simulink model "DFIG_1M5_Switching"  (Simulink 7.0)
settings: Solver=ode45  SolverMode=SingleTasking  StartTime=0  StopTime=Tstop  FixedStep=0,000005  MaxStep=0.001  RelTol=1e-3  AbsTol=1e-6
InitFcn:
  | DFIG_init_sw
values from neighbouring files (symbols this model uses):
  gearbox = 75.7098    [DFIG_init_simp.m]    (also in DFIG_init_sw.m)
  ki_i = 0.003    [DFIG_init_simp.m]    (also in DFIG_init_sw.m)
  kp_i = 0.00003    (= 3e-05)    [DFIG_init_simp.m]    (also in DFIG_init_sw.m)
  L = 0.6e-3    (= 0.0006)    [DFIG_init_simp.m]    (also in DFIG_init_sw.m)
  R = 35    [DFIG_init_simp.m]    (also in DFIG_init_sw.m)
  TSR_opt = 8    [DFIG_init_simp.m]    (also in DFIG_init_sw.m)
  Tswitch = 0.2    [DFIG_init_simp.m]    (also in DFIG_init_sw.m)
  Vw1 = 10.5    [DFIG_init_simp.m]    (also in DFIG_init_sw.m)
  Vw2 = 8    [DFIG_init_simp.m]    (also in DFIG_init_sw.m)
  zp = 2    [DFIG_init_simp.m]    (also in DFIG_init_sw.m)
undefined symbols (not defined in the file or in its folder): carrier, Natural, plecsedit, starts, with
libraries: plecslib x10, plecslib_extras x7, simulink x2

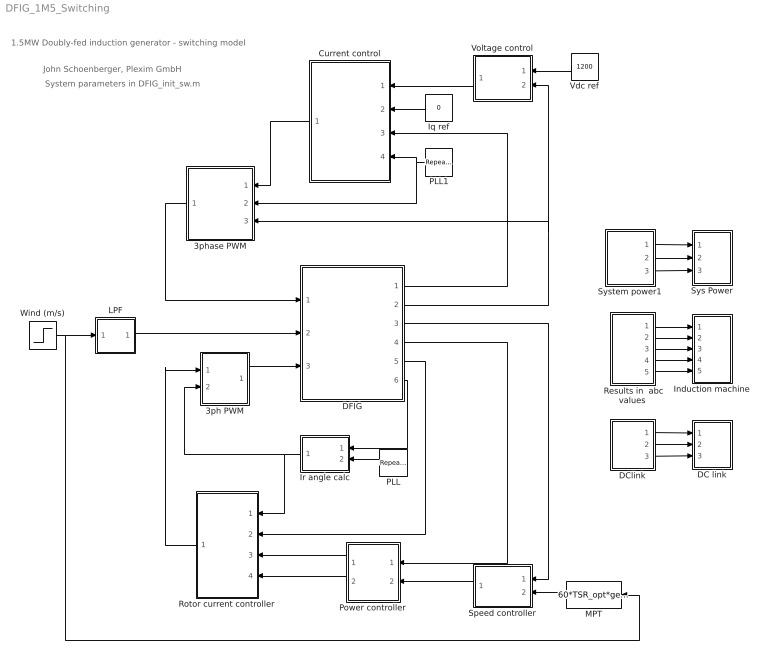
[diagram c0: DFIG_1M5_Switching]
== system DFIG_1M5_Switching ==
  note: John Schoenberger, Plexim GmbH
  note: 1.5MW Doubly-fed induction generator - switching model
  note: System parameters in DFIG_init_sw.m
  " Results in  abc values" : Subsystem
  3ph PWM : Subsystem
  3phase PWM : Subsystem  Orientation=left
  Current control : Subsystem  Orientation=left
  DC link : Subsystem  LoadFcn=plecsedit('sl', 300);  StartFcn=plecsedit('sl', 308);  StopFcn=plecsedit('sl', 309);  mask{Settings=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}
      mask init:
      | plecsedit('sl', 315);
  DClink : Subsystem
  DFIG : Subsystem  LoadFcn=plecsedit('sl', 200);  InitFcn=plecsedit('sl', 214);  StartFcn=plecsedit('sl', 208);  StopFcn=plecsedit('sl', 209);
  Induction machine : Subsystem  LoadFcn=plecsedit('sl', 300);  StartFcn=plecsedit('sl', 308);  StopFcn=plecsedit('sl', 309);  mask{Settings=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}
      mask init:
      | plecsedit('sl', 315);
  Iq ref : Constant  Orientation=left  Value=0  OutDataType=sfix(16)  OutScaling=2^0
  Ir angle calc : Subsystem  Orientation=left
  LPF : Subsystem  mask{tau=0.2, y0=Vw1}
      mask prompts: tau "Time constant"; y0 "Initial output"
  MPT : Fcn  Orientation=left  Expr=60*TSR_opt*gearbox*u(1)/(2*pi*R)
  PLL : simulink/Sources/Repeating Sequence  Orientation=left  SystemSampleTime=-1  rep_seq_t=[0 0.02]  rep_seq_y=[-pi/2 3/2*pi]
  PLL1 : simulink/Sources/Repeating Sequence  Orientation=left  SystemSampleTime=-1  rep_seq_t=[0 0.02]  rep_seq_y=[-pi/2 3/2*pi]
  Power controller : Subsystem  Orientation=left
  Rotor current controller : Subsystem  Orientation=left
  Speed controller : Subsystem  Orientation=left
  Sys Power : Subsystem  LoadFcn=plecsedit('sl', 300);  StartFcn=plecsedit('sl', 308);  StopFcn=plecsedit('sl', 309);  mask{Settings=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}
      mask init:
      | plecsedit('sl', 315);
  System power1 : Subsystem
  Vdc ref : Constant  Orientation=left  Value=1200  OutDataType=sfix(16)  OutScaling=2^0
  Voltage control : Subsystem  Orientation=left
  Wind (m/s) : Step  Time=Tswitch  Before=Vw1  After=Vw2  SampleTime=0
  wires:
  DFIG/4(P,Q) -> Power controller/1(S)
  DFIG/5(Ir 2) -> Rotor current controller/2(Ir2)
  DFIG/6(th r) -> Ir angle calc/1(th r)
  Ir angle calc/1(th Ir) -> 3ph PWM/2(theta), Rotor current controller/1(theta)
  " Results in  abc values"/1(Irabc) -> Induction machine/1(1)
  " Results in  abc values"/2(Isabc) -> Induction machine/2(2)
  " Results in  abc values"/3(Vrabc) -> Induction machine/3(3)
  " Results in  abc values"/4(speed) -> Induction machine/4(4)
  " Results in  abc values"/5(Torque) -> Induction machine/5(5)
  DClink/1(Idc in) -> DC link/1(1)
  DClink/2(Vdc) -> DC link/2(2)
  DClink/3(Pdc in) -> DC link/3(3)
  Wind (m/s)/1 -> MPT/1, LPF/1(Vw)
  LPF/1(Vw') -> DFIG/2(Vwind)
  Power controller/1(Irq*) -> Rotor current controller/3(Irq*)
  Power controller/2(Ird*) -> Rotor current controller/4(Ird*)
  PLL/1 -> Ir angle calc/2(th 50Hz)
  System power1/1(Stator PQ) -> Sys Power/1(1)
  System power1/2(Rotor PQ) -> Sys Power/2(2)
  System power1/3(Sys PQ) -> Sys Power/3(3)
  Speed controller/1(P*) -> Power controller/2(P*)
  DFIG/3(rpm) -> Speed controller/1(rpm)
  MPT/1 -> Speed controller/2(rpm*)
  3ph PWM/1(Sabc) -> DFIG/3(S2)
  Voltage control/1(Id*) -> Current control/1(Id*)
  3phase PWM/1(SW) -> DFIG/1(S1)
  Current control/1(Vdq*) -> 3phase PWM/1(Vdq*)
  Iq ref/1 -> Current control/2(Iq*)
  Vdc ref/1 -> Voltage control/1(Vdc*)
  DFIG/2(Vdc) -> 3phase PWM/3(Vdc), Voltage control/2(Vdc)
  DFIG/1(ir 1) -> Current control/3(Igrid)
  PLL1/1 -> 3phase PWM/2(theta), Current control/4(PLL)
  Rotor current controller/1(Vr dq*) -> 3ph PWM/1(Vr dq*)

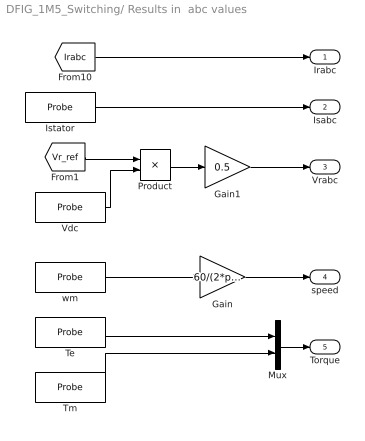
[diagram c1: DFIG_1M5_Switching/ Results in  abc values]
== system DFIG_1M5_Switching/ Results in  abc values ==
  Gain : Gain  Gain=60/(2*pi)  ParameterDataType=sfix(16)  ParameterScaling=2^0  OutDataType=sfix(16)  OutScaling=2^0
  Gain1 : Gain  Gain=0.5  ParameterDataType=sfix(16)  ParameterScaling=2^0  OutDataType=sfix(16)  OutScaling=2^0
  Istator : plecslib/Probe  SystemSampleTime=-1  tagno=18
  Mux : Mux  Inputs=2
  Product : Product  OutDataType=sfix(16)  OutScaling=2^0
  Te : plecslib/Probe  SystemSampleTime=-1  tagno=1
  Tm : plecslib/Probe  SystemSampleTime=-1  tagno=5
  Vdc : plecslib/Probe  SystemSampleTime=-1  tagno=4
  wm : plecslib/Probe  SystemSampleTime=-1  tagno=2
  Irabc : Outport
  Isabc : Outport  Port=2
  Vrabc : Outport  Port=3
  speed : Outport  Port=4
  Torque : Outport  Port=5
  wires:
  Gain/1 -> speed/1
  Istator/1 -> Isabc/1
  [Irabc] -> Irabc/1
  Product/1 -> Gain1/1
  Te/1 -> Mux/1
  Tm/1 -> Mux/2
  Mux/1 -> Torque/1
  wm/1 -> Gain/1
  [Vr_ref] -> Product/1
  Vdc/1 -> Product/2
  Gain1/1 -> Vrabc/1

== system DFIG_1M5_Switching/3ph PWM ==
  Vr dq* : Inport  OutDataType=sfix(16)  OutScaling=2^0
  theta : Inport  Port=2  OutDataType=sfix(16)  OutScaling=2^0
  Modulator : plecslib_extras/Modulators/Symmetrical PWM  SystemSampleTime=-1  sampling=Natural (carrier starts with 0)  fc=fs  offset=0
  RRF->3ph : plecslib_extras/Transformations/RRF->3ph  SystemSampleTime=-1
  Sabc : Outport
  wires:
  Modulator/1 -> Sabc/1
  theta/1 -> RRF->3ph/2
  RRF->3ph/1 -> [Vr_ref], Modulator/1
  Vr dq*/1 -> RRF->3ph/1

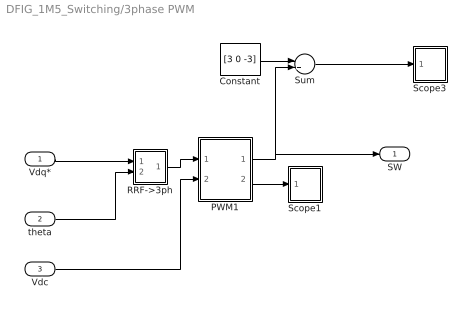
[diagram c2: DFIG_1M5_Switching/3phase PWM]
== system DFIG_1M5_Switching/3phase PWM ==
  Vdq* : Inport  OutDataType=sfix(16)  OutScaling=2^0
  theta : Inport  Port=2  OutDataType=sfix(16)  OutScaling=2^0
  Vdc : Inport  Port=3  OutDataType=sfix(16)  OutScaling=2^0
  Constant : Constant  Value=[3 0 -3]  OutDataType=sfix(16)  OutScaling=2^0
  PWM1 : Subsystem
  RRF->3ph : Subsystem
  Scope1 : Subsystem  LoadFcn=plecsedit('sl', 300);  StartFcn=plecsedit('sl', 308);  StopFcn=plecsedit('sl', 309);  mask{Settings=AAAAAQAAAAEAAAAAAAAAAAEAAAAAAAAAAP///////////////wD/////AQAAAAAAAAAAP/AAAAAAAAAAAAAA/////wAAAAD/////AAAAAA==}
      mask init:
      | plecsedit('sl', 315);
  Scope3 : Subsystem  LoadFcn=plecsedit('sl', 300);  StartFcn=plecsedit('sl', 308);  StopFcn=plecsedit('sl', 309);  mask{Settings=AAAAAQAAAAEAAAAAAAAAAAEAAAAAAAAAAP///////////////wD/////AQAAAAAAAAAAP/AAAAAAAAAAAAAA/////wAAAAD/////AAAAAA==}
      mask init:
      | plecsedit('sl', 315);
  Sum : Sum  OutDataType=sfix(16)  OutScaling=2^0
  SW : Outport  OutDataType=sfix(16)  OutScaling=2^0
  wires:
  RRF->3ph/1(abc) -> PWM1/1(m)
  PWM1/2(m_out) -> Scope1/1(1)
  theta/1 -> RRF->3ph/2(phi)
  Vdc/1 -> PWM1/2(v_dc)
  PWM1/1(pulses) -> SW/1, Sum/2
  Constant/1 -> Sum/1
  Sum/1 -> Scope3/1(1)
  Vdq*/1 -> RRF->3ph/1(dq)

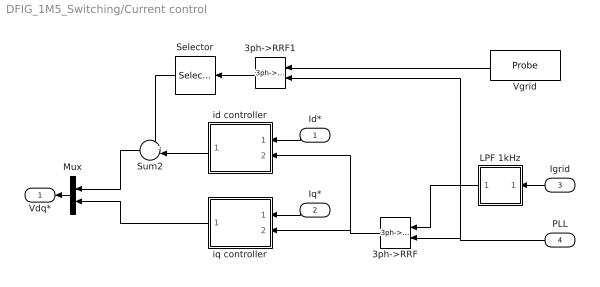
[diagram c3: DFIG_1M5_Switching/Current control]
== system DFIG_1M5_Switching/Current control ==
  Id* : Inport  Orientation=left
  Iq* : Inport  Orientation=left  Port=2
  Igrid : Inport  Orientation=left  Port=3  OutDataType=sfix(16)  OutScaling=2^0
  PLL : Inport  Orientation=left  Port=4  OutDataType=sfix(16)  OutScaling=2^0
  3ph->RRF : plecslib_extras/Transformations/3ph->RRF  Orientation=left  SystemSampleTime=-1
  3ph->RRF1 : plecslib_extras/Transformations/3ph->RRF  Orientation=left  SystemSampleTime=-1
  LPF 1kHz : Subsystem  Orientation=left  mask{tau=1.6e-4, y0=0}
      mask prompts: tau "Time constant"; y0 "Initial output"
  Mux : Mux  Orientation=left  Inputs=2
  Selector : Selector  Orientation=left  InputPortWidth=2  IndexOptions=Index vector (dialog)  Indices=1  OutputSizes=1
  Sum2 : Sum  Orientation=left  Inputs=+-|  OutDataType=sfix(16)  OutScaling=2^0
  Vgrid : plecslib/Probe  Orientation=left  SystemSampleTime=-1  tagno=17
  id controller : Subsystem  Orientation=left
  iq controller : Subsystem  Orientation=left
  Vdq* : Outport  Orientation=left
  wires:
  id controller/1(Vd*) -> Sum2/2
  Selector/1 -> Sum2/1
  3ph->RRF1/1 -> Selector/1
  Id*/1 -> id controller/1(id ref)
  Iq*/1 -> iq controller/1(iq ref)
  PLL/1 -> 3ph->RRF/2, 3ph->RRF1/2
  Igrid/1 -> LPF 1kHz/1(I)
  Vgrid/1 -> 3ph->RRF1/1
  Mux/1 -> Vdq*/1
  Sum2/1 -> Mux/1
  iq controller/1(Vq*) -> Mux/2
  LPF 1kHz/1(Ifilt) -> 3ph->RRF/1
  3ph->RRF/1 -> id controller/2(i), iq controller/2(i)

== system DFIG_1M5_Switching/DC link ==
  1 : Inport  OutDataType=sfix(16)  OutScaling=2^0
  2 : Inport  Port=2  OutDataType=sfix(16)  OutScaling=2^0
  3 : Inport  Port=3  OutDataType=sfix(16)  OutScaling=2^0
  " InputMux " : Subsystem
  " S-Function " : S-Function  FunctionName=plecsedit
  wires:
  " InputMux "/1(Out) -> " S-Function "/1
  1/1 -> " InputMux "/1(In1)
  2/1 -> " InputMux "/2(In2)
  3/1 -> " InputMux "/3(In3)

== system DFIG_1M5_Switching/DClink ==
  DC current from grid converter : plecslib/Probe  SystemSampleTime=-1  tagno=14
  Product : Product  OutDataType=sfix(16)  OutScaling=2^0
  vdc : plecslib/Probe  SystemSampleTime=-1  tagno=15
  Idc in : Outport
  Vdc : Outport  Port=2
  Pdc in : Outport  Port=3
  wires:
  DC current from grid converter/1 -> Idc in/1, Product/1
  vdc/1 -> Vdc/1, Product/2
  Product/1 -> Pdc in/1

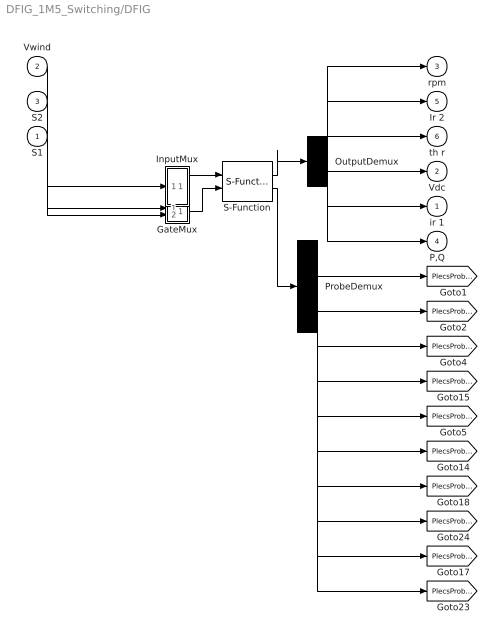
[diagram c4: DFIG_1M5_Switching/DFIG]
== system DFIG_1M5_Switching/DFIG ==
  S1 : Inport  PortDimensions=3
  Vwind : Inport  Port=2  PortDimensions=1  OutDataType=sfix(16)  OutScaling=2^0
  S2 : Inport  Port=3  PortDimensions=3  OutDataType=sfix(16)  OutScaling=2^0
  " GateMux " : Subsystem
  " InputMux " : Subsystem
  " OutputDemux " : Demux  Outputs=[ 1 3 1 1 3 2 ]
  " ProbeDemux " : Demux  Outputs=[ 1 1 1 1 1 1 3 3 3 3 ]
  " S-Function " : S-Function  FunctionName=plecsedit
  ir 1 : Outport  PortDimensions=3
  Vdc : Outport  Port=2  PortDimensions=1  OutDataType=sfix(16)  OutScaling=2^0
  rpm : Outport  Port=3  PortDimensions=1  OutDataType=sfix(16)  OutScaling=2^0
  P,Q : Outport  Port=4  PortDimensions=2
  Ir 2 : Outport  Port=5  PortDimensions=3  OutDataType=sfix(16)  OutScaling=2^0
  th r : Outport  Port=6  PortDimensions=1  OutDataType=sfix(16)  OutScaling=2^0
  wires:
  " S-Function "/2 -> " ProbeDemux "/1
  " GateMux "/1(Out) -> " S-Function "/2
  " InputMux "/1(Out) -> " S-Function "/1
  " S-Function "/1 -> " OutputDemux "/1
  Vwind/1 -> " InputMux "/1(In1)
  S2/1 -> " GateMux "/1(In1)
  S1/1 -> " GateMux "/2(In2)
  " OutputDemux "/1 -> rpm/1
  " OutputDemux "/2 -> Ir 2/1
  " OutputDemux "/3 -> th r/1
  " OutputDemux "/4 -> Vdc/1
  " OutputDemux "/5 -> ir 1/1
  " OutputDemux "/6 -> P,Q/1
  " ProbeDemux "/1 -> [PlecsProbe1]
  " ProbeDemux "/2 -> [PlecsProbe2]
  " ProbeDemux "/3 -> [PlecsProbe4]
  " ProbeDemux "/4 -> [PlecsProbe15]
  " ProbeDemux "/5 -> [PlecsProbe5]
  " ProbeDemux "/6 -> [PlecsProbe14]
  " ProbeDemux "/7 -> [PlecsProbe18]
  " ProbeDemux "/8 -> [PlecsProbe24]
  " ProbeDemux "/9 -> [PlecsProbe17]
  " ProbeDemux "/10 -> [PlecsProbe23]

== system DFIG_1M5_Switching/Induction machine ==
  1 : Inport  OutDataType=sfix(16)  OutScaling=2^0
  2 : Inport  Port=2  OutDataType=sfix(16)  OutScaling=2^0
  3 : Inport  Port=3  OutDataType=sfix(16)  OutScaling=2^0
  4 : Inport  Port=4  OutDataType=sfix(16)  OutScaling=2^0
  5 : Inport  Port=5  OutDataType=sfix(16)  OutScaling=2^0
  " InputMux " : Subsystem
  " S-Function " : S-Function  FunctionName=plecsedit
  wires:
  " InputMux "/1(Out) -> " S-Function "/1
  1/1 -> " InputMux "/1(In1)
  2/1 -> " InputMux "/2(In2)
  3/1 -> " InputMux "/3(In3)
  4/1 -> " InputMux "/4(In4)
  5/1 -> " InputMux "/5(In5)

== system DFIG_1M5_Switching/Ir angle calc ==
  th r : Inport  OutDataType=sfix(16)  OutScaling=2^0
  th 50Hz : Inport  Port=2  OutDataType=sfix(16)  OutScaling=2^0
  Gain : Gain  Gain=zp  ParameterDataType=sfix(16)  ParameterScaling=2^0  OutDataType=sfix(16)  OutScaling=2^0
  Sum1 : Sum  Inputs=+-  OutDataType=sfix(16)  OutScaling=2^0
  th Ir : Outport
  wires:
  th r/1 -> Gain/1
  th 50Hz/1 -> Sum1/1
  Sum1/1 -> th Ir/1
  Gain/1 -> Sum1/2

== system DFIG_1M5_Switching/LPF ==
  Vw : Inport  OutDataType=sfix(16)  OutScaling=2^0
  Gain : Gain  Gain=1/tau  ParameterDataType=sfix(16)  ParameterScaling=2^0  OutDataType=sfix(16)  OutScaling=2^0
  Integrator : Integrator  InitialCondition=y0
  Subtract : Sum  Inputs=+-  OutDataType=sfix(16)  OutScaling=2^-10
  Vw' : Outport  OutDataType=sfix(16)  OutScaling=2^0
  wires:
  Integrator/1 -> Vw'/1, Subtract/2
  Vw/1 -> Subtract/1
  Subtract/1 -> Gain/1
  Gain/1 -> Integrator/1

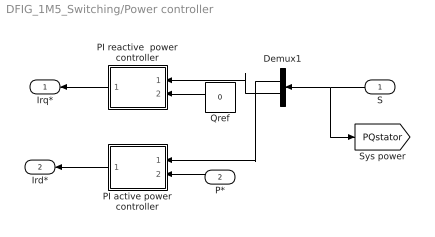
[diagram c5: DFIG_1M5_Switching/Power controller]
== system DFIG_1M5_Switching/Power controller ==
  S : Inport  Orientation=left  OutDataType=sfix(16)  OutScaling=2^0
  P* : Inport  Orientation=left  Port=2  OutDataType=sfix(16)  OutScaling=2^0
  Demux1 : Demux  Orientation=left  Outputs=2
  PI active power controller : Subsystem  Orientation=left
  PI reactive  power controller : Subsystem  Orientation=left
  Qref : Constant  Orientation=left  Value=0  OutDataType=sfix(16)  OutScaling=2^0
  Irq* : Outport  Orientation=left  OutDataType=sfix(16)  OutScaling=2^0
  Ird* : Outport  Orientation=left  Port=2  OutDataType=sfix(16)  OutScaling=2^0
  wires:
  Demux1/2 -> PI reactive  power controller/1(Q)
  Demux1/1 -> PI active power controller/1(P)
  S/1 -> [PQstator], Demux1/1
  P*/1 -> PI active power controller/2(Pref)
  PI active power controller/1(Irdref) -> Ird*/1
  PI reactive  power controller/1(Irqref) -> Irq*/1
  Qref/1 -> PI reactive  power controller/2(Qref)

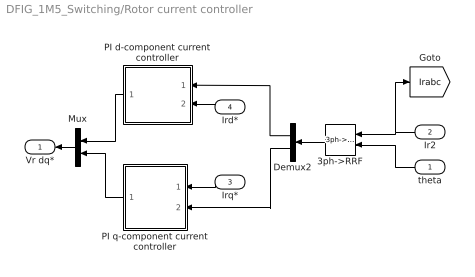
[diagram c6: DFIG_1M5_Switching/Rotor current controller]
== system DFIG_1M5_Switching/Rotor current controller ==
  theta : Inport  Orientation=left  OutDataType=sfix(16)  OutScaling=2^0
  Ir2 : Inport  Orientation=left  Port=2  OutDataType=sfix(16)  OutScaling=2^0
  Irq* : Inport  Orientation=left  Port=3  OutDataType=sfix(16)  OutScaling=2^0
  Ird* : Inport  Orientation=left  Port=4  OutDataType=sfix(16)  OutScaling=2^0
  3ph->RRF : plecslib_extras/Transformations/3ph->RRF  Orientation=left  SystemSampleTime=-1
  Demux2 : Demux  Orientation=left  Outputs=2
  Mux : Mux  Orientation=left  Inputs=2
  PI d-component current controller : Subsystem  Orientation=left
  PI q-component current controller : Subsystem  Orientation=left
  Vr dq* : Outport  Orientation=left  OutDataType=sfix(16)  OutScaling=2^0
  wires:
  Demux2/2 -> PI q-component current controller/2(Irq)
  Demux2/1 -> PI d-component current controller/1(Ird)
  theta/1 -> 3ph->RRF/2
  Ir2/1 -> [Irabc], 3ph->RRF/1
  3ph->RRF/1 -> Demux2/1
  PI q-component current controller/1(Vrq) -> Mux/2
  PI d-component current controller/1(Vrd) -> Mux/1
  Mux/1 -> Vr dq*/1
  Ird*/1 -> PI d-component current controller/2(Irdref)
  Irq*/1 -> PI q-component current controller/1(Irqref)

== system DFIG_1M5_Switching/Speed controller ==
  rpm : Inport  Orientation=left  OutDataType=sfix(16)  OutScaling=2^0
  rpm* : Inport  Orientation=left  Port=2  OutDataType=sfix(16)  OutScaling=2^0
  Integrator : Integrator  Orientation=left  UpperSaturationLimit=5000  LowerSaturationLimit=-5000
  Ki : Gain  Orientation=left  Gain=1500  ParameterDataType=sfix(16)  ParameterScaling=2^0  OutDataType=sfix(16)  OutScaling=2^0
  Kp : Gain  Orientation=left  Gain=750  ParameterDataType=sfix(16)  ParameterScaling=2^0  OutDataType=sfix(16)  OutScaling=2^0
  Sum1 : Sum  Orientation=left  OutDataType=sfix(16)  OutScaling=2^0
  Sum3 : Sum  Orientation=left  Inputs=+-  OutDataType=sfix(16)  OutScaling=2^0
  P* : Outport  Orientation=left
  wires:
  rpm/1 -> Sum3/2
  rpm*/1 -> Sum3/1
  Integrator/1 -> Sum1/2
  Sum1/1 -> P*/1
  Kp/1 -> Sum1/1
  Ki/1 -> Integrator/1
  Sum3/1 -> Ki/1, Kp/1

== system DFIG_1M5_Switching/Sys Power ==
  1 : Inport  OutDataType=sfix(16)  OutScaling=2^0
  2 : Inport  Port=2  OutDataType=sfix(16)  OutScaling=2^0
  3 : Inport  Port=3  OutDataType=sfix(16)  OutScaling=2^0
  " InputMux " : Subsystem
  " S-Function " : S-Function  FunctionName=plecsedit
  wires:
  " InputMux "/1(Out) -> " S-Function "/1
  1/1 -> " InputMux "/1(In1)
  2/1 -> " InputMux "/2(In2)
  3/1 -> " InputMux "/3(In3)

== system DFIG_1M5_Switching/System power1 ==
  3 phase  P & Q1 : Subsystem  DialogController=PMDialogs.PMDefaultMaskDlg
  Rotor current : plecslib/Probe  SystemSampleTime=-1  tagno=24
  Sum of Elements : Sum  OutDataType=sfix(16)  OutScaling=2^-10
  Sys voltage : plecslib/Probe  SystemSampleTime=-1  tagno=23
  Stator PQ : Outport
  Rotor PQ : Outport  Port=2
  Sys PQ : Outport  Port=3
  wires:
  Sum of Elements/1 -> Sys PQ/1
  [PQstator] -> Sum of Elements/1, Stator PQ/1
  Rotor current/1 -> 3 phase  P & Q1/2(Iabc)
  Sys voltage/1 -> 3 phase  P & Q1/1(Vabc)
  3 phase  P & Q1/1(PQ) -> Sum of Elements/2, Rotor PQ/1

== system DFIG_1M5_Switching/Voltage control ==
  Vdc* : Inport  Orientation=left  PortDimensions=1  OutDataType=sfix(16)  OutScaling=2^0
  Vdc : Inport  Orientation=left  Port=2  PortDimensions=1  OutDataType=sfix(16)  OutScaling=2^0
  I : Gain  Orientation=left  Gain=20  ParameterDataType=sfix(16)  ParameterScaling=2^0  OutDataType=sfix(16)  OutScaling=2^0
  Integrator : Integrator  Orientation=left
  P : Gain  Orientation=left  Gain=2  ParameterDataType=sfix(16)  ParameterScaling=2^0  OutDataType=sfix(16)  OutScaling=2^0
  Sum1 : Sum  Orientation=left  OutDataType=sfix(16)  OutScaling=2^0
  Sum2 : Sum  Orientation=left  Inputs=+-  OutDataType=sfix(16)  OutScaling=2^0
  Id* : Outport  Orientation=left  OutDataType=sfix(16)  OutScaling=2^0
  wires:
  Integrator/1 -> Sum1/2
  Vdc/1 -> Sum2/2
  Vdc*/1 -> Sum2/1
  Sum2/1 -> I/1, P/1
  Sum1/1 -> Id*/1
  I/1 -> Integrator/1
  P/1 -> Sum1/1

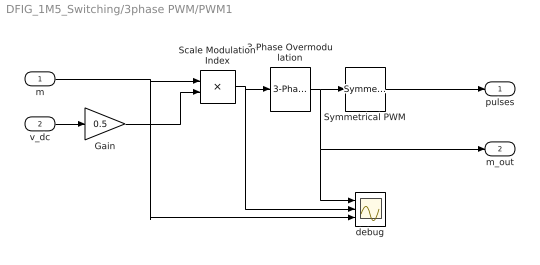
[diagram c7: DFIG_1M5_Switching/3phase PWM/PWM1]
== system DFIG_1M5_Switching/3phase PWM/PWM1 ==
  m : Inport  OutDataType=sfix(16)  OutScaling=2^0
  v_dc : Inport  Port=2  OutDataType=sfix(16)  OutScaling=2^0
  3-Phase Overmodulation : plecslib_extras/Modulators/3-Phase Overmodulation  SystemSampleTime=-1
  Gain : Gain  Gain=0.5  ParameterDataType=sfix(16)  ParameterScaling=2^0  OutDataType=sfix(16)  OutScaling=2^0
  Scale Modulation Index : Product  Inputs=*/  OutDataType=sfix(16)  OutScaling=2^0
  Symmetrical PWM : plecslib_extras/Modulators/Symmetrical PWM  SystemSampleTime=-1  sampling=Natural (carrier starts with 0)  fc=fs1  offset=0
  debug : Scope  NumInputPorts=3
  pulses : Outport  OutDataType=sfix(16)  OutScaling=2^0
  m_out : Outport  Port=2  OutDataType=sfix(16)  OutScaling=2^0
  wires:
  Symmetrical PWM/1 -> pulses/1
  v_dc/1 -> Gain/1
  Scale Modulation Index/1 -> 3-Phase Overmodulation/1, debug/2
  m/1 -> Scale Modulation Index/1, debug/3
  Gain/1 -> Scale Modulation Index/2
  3-Phase Overmodulation/1 -> Symmetrical PWM/1, debug/1, m_out/1

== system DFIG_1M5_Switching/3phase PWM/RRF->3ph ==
  dq : Inport  PortDimensions=2  OutDataType=sfix(16)  OutScaling=2^0
  phi : Inport  Port=2  PortDimensions=1  OutDataType=sfix(16)  OutScaling=2^0
  Mux1 : Mux  Inputs=2
  Mux2 : Mux  Inputs=3
  dq->a : Fcn  Expr=u[1]*cos(u[3])-u[2]*sin(u[3])
  dq->b : Fcn  Expr=u[1]*cos(u[3]-2*pi/3)-u[2]*sin(u[3]-2*pi/3)
  dq->c : Fcn  Expr=u[1]*cos(u[3]+2*pi/3)-u[2]*sin(u[3]+2*pi/3)
  abc : Outport  OutDataType=sfix(16)  OutScaling=2^0
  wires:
  dq->c/1 -> Mux2/3
  Mux2/1 -> abc/1
  dq->b/1 -> Mux2/2
  dq->a/1 -> Mux2/1
  Mux1/1 -> dq->c/1, dq->b/1, dq->a/1
  dq/1 -> Mux1/1
  phi/1 -> Mux1/2

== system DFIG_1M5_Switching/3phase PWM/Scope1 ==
  1 : Inport  OutDataType=sfix(16)  OutScaling=2^0
  " InputMux " : Subsystem
  " S-Function " : S-Function  FunctionName=plecsedit
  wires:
  1/1 -> " InputMux "/1(In1)
  " InputMux "/1(Out) -> " S-Function "/1

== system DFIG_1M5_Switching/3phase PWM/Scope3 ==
  1 : Inport  OutDataType=sfix(16)  OutScaling=2^0
  " InputMux " : Subsystem
  " S-Function " : S-Function  FunctionName=plecsedit
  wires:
  " InputMux "/1(Out) -> " S-Function "/1
  1/1 -> " InputMux "/1(In1)

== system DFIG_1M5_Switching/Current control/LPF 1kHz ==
  I : Inport  OutDataType=sfix(16)  OutScaling=2^0
  Gain : Gain  Gain=1/tau  ParameterDataType=sfix(16)  ParameterScaling=2^0  OutDataType=sfix(16)  OutScaling=2^0
  Integrator : Integrator  InitialCondition=y0
  Subtract : Sum  Inputs=+-  OutDataType=sfix(16)  OutScaling=2^-10
  Ifilt : Outport  OutDataType=sfix(16)  OutScaling=2^0
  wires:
  Gain/1 -> Integrator/1
  Subtract/1 -> Gain/1
  I/1 -> Subtract/1
  Integrator/1 -> Subtract/2, Ifilt/1

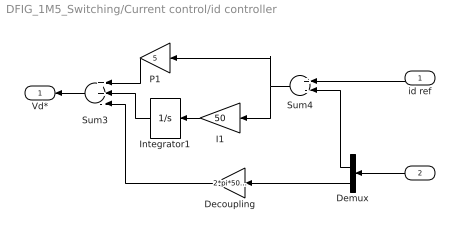
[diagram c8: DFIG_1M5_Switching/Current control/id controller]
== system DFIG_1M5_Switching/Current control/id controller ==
  id ref : Inport  Orientation=left  OutDataType=sfix(16)  OutScaling=2^0
  i : Inport  Orientation=left  Port=2  PortDimensions=2  OutDataType=sfix(16)  OutScaling=2^0
  Decoupling : Gain  Orientation=left  Gain=2*pi*50*L  Multiplication=Matrix(K*u)  ParameterDataType=sfix(16)  ParameterScaling=2^0  OutDataType=sfix(16)  OutScaling=2^0
  Demux : Demux  Orientation=left  Outputs=2
  I1 : Gain  Orientation=left  Gain=50  ParameterDataType=sfix(16)  ParameterScaling=2^0  OutDataType=sfix(16)  OutScaling=2^0
  Integrator1 : Integrator  Orientation=left
  P1 : Gain  Orientation=left  Gain=5  ParameterDataType=sfix(16)  ParameterScaling=2^0  OutDataType=sfix(16)  OutScaling=2^0
  Sum3 : Sum  Orientation=left  Inputs=++-  OutDataType=sfix(16)  OutScaling=2^0
  Sum4 : Sum  Orientation=left  Inputs=+-  OutDataType=sfix(16)  OutScaling=2^0
  Vd* : Outport  Orientation=left  OutDataType=sfix(16)  OutScaling=2^0
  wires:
  Sum3/1 -> Vd*/1
  i/1 -> Demux/1
  Demux/2 -> Decoupling/1
  Demux/1 -> Sum4/2
  Decoupling/1 -> Sum3/3
  id ref/1 -> Sum4/1
  Integrator1/1 -> Sum3/2
  Sum4/1 -> P1/1, I1/1
  I1/1 -> Integrator1/1
  P1/1 -> Sum3/1

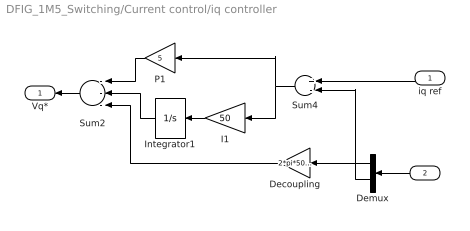
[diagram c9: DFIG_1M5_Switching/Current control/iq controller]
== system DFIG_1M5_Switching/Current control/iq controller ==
  iq ref : Inport  Orientation=left  OutDataType=sfix(16)  OutScaling=2^0
  i : Inport  Orientation=left  Port=2  PortDimensions=2  OutDataType=sfix(16)  OutScaling=2^0
  Decoupling : Gain  Orientation=left  Gain=2*pi*50*L  Multiplication=Matrix(K*u)  ParameterDataType=sfix(16)  ParameterScaling=2^0  OutDataType=sfix(16)  OutScaling=2^0
  Demux : Demux  Orientation=left  Outputs=2
  I1 : Gain  Orientation=left  Gain=50  ParameterDataType=sfix(16)  ParameterScaling=2^0  OutDataType=sfix(16)  OutScaling=2^0
  Integrator1 : Integrator  Orientation=left
  P1 : Gain  Orientation=left  Gain=5  ParameterDataType=sfix(16)  ParameterScaling=2^0  OutDataType=sfix(16)  OutScaling=2^0
  Sum2 : Sum  Orientation=left  Inputs=---  OutDataType=sfix(16)  OutScaling=2^0
  Sum4 : Sum  Orientation=left  Inputs=+-  OutDataType=sfix(16)  OutScaling=2^0
  Vq* : Outport  Orientation=left  OutDataType=sfix(16)  OutScaling=2^0
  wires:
  Demux/1 -> Decoupling/1
  Demux/2 -> Sum4/2
  Sum2/1 -> Vq*/1
  P1/1 -> Sum2/1
  i/1 -> Demux/1
  Decoupling/1 -> Sum2/3
  iq ref/1 -> Sum4/1
  Integrator1/1 -> Sum2/2
  Sum4/1 -> I1/1, P1/1
  I1/1 -> Integrator1/1

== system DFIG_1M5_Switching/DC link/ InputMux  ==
  In1 : Inport  OutDataType=sfix(16)  OutScaling=2^0
  In2 : Inport  Port=2  OutDataType=sfix(16)  OutScaling=2^0
  In3 : Inport  Port=3  OutDataType=sfix(16)  OutScaling=2^0
  Convert1 : DataTypeConversion  OutDataType=sfix(16)  OutScaling=2^0
  Convert2 : DataTypeConversion  OutDataType=sfix(16)  OutScaling=2^0
  Convert3 : DataTypeConversion  OutDataType=sfix(16)  OutScaling=2^0
  Mux : Mux  Inputs=3
  Out : Outport  OutDataType=sfix(16)  OutScaling=2^0
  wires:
  Mux/1 -> Out/1
  In1/1 -> Convert1/1
  In2/1 -> Convert2/1
  In3/1 -> Convert3/1
  Convert1/1 -> Mux/1
  Convert2/1 -> Mux/2
  Convert3/1 -> Mux/3

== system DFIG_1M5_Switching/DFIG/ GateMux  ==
  In1 : Inport
  In2 : Inport  Port=2
  Convert1 : DataTypeConversion
  Convert2 : DataTypeConversion
  Mux : Mux  Inputs=[ 3 3 ]
  Out : Outport
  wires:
  Mux/1 -> Out/1
  In1/1 -> Convert1/1
  In2/1 -> Convert2/1
  Convert1/1 -> Mux/1
  Convert2/1 -> Mux/2

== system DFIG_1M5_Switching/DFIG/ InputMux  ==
  In1 : Inport  OutDataType=sfix(16)  OutScaling=2^0
  Convert1 : DataTypeConversion  OutDataType=sfix(16)  OutScaling=2^0
  Mux : Mux  Inputs=[ 1 ]
  Out : Outport  OutDataType=sfix(16)  OutScaling=2^0
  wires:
  Mux/1 -> Out/1
  In1/1 -> Convert1/1
  Convert1/1 -> Mux/1

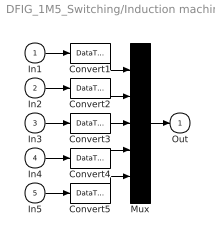
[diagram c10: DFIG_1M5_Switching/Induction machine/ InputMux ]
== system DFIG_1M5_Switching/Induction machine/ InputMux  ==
  In1 : Inport  OutDataType=sfix(16)  OutScaling=2^0
  In2 : Inport  Port=2  OutDataType=sfix(16)  OutScaling=2^0
  In3 : Inport  Port=3  OutDataType=sfix(16)  OutScaling=2^0
  In4 : Inport  Port=4  OutDataType=sfix(16)  OutScaling=2^0
  In5 : Inport  Port=5  OutDataType=sfix(16)  OutScaling=2^0
  Convert{1..5} (5 alike) : DataTypeConversion  OutDataType=sfix(16)  OutScaling=2^0
  Mux : Mux  Inputs=5
  Out : Outport  OutDataType=sfix(16)  OutScaling=2^0
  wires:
  Mux/1 -> Out/1
  In1/1 -> Convert1/1
  In2/1 -> Convert2/1
  In3/1 -> Convert3/1
  In4/1 -> Convert4/1
  In5/1 -> Convert5/1
  Convert1/1 -> Mux/1
  Convert2/1 -> Mux/2
  Convert3/1 -> Mux/3
  Convert4/1 -> Mux/4
  Convert5/1 -> Mux/5

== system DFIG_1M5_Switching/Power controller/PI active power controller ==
  P : Inport  Orientation=left  OutDataType=sfix(16)  OutScaling=2^0
  Pref : Inport  Orientation=left  Port=2  OutDataType=sfix(16)  OutScaling=2^0
  Gain : Gain  Orientation=left  Gain=0.0002  ParameterDataType=sfix(16)  ParameterScaling=2^0  OutDataType=sfix(16)  OutScaling=2^0
  Gain1 : Gain  Orientation=left  Gain=0.05  ParameterDataType=sfix(16)  ParameterScaling=2^0  OutDataType=sfix(16)  OutScaling=2^0
  Integrator2 : Integrator  Orientation=left
  Sum2 : Sum  Orientation=left  Inputs=|+-  OutDataType=sfix(16)  OutScaling=2^0
  Sum3 : Sum  Orientation=left  Inputs=+-  OutDataType=sfix(16)  OutScaling=2^0
  Irdref : Outport  Orientation=left
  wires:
  Gain1/1 -> Integrator2/1
  Gain/1 -> Sum2/1
  Sum2/1 -> Irdref/1
  Pref/1 -> Sum3/1
  P/1 -> Sum3/2
  Sum3/1 -> Gain1/1, Gain/1
  Integrator2/1 -> Sum2/2

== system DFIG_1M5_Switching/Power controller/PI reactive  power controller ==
  Q : Inport  Orientation=left  OutDataType=sfix(16)  OutScaling=2^0
  Qref : Inport  Orientation=left  Port=2  OutDataType=sfix(16)  OutScaling=2^0
  -1/(sqrt(3)*Vpp) : Gain  Orientation=left  Gain=0.0002  ParameterDataType=sfix(16)  ParameterScaling=2^0  OutDataType=sfix(16)  OutScaling=2^0
  Gain6 : Gain  Orientation=left  Gain=0.005  ParameterDataType=sfix(16)  ParameterScaling=2^0  OutDataType=sfix(16)  OutScaling=2^0
  Integrator2 : Integrator  Orientation=left
  Sum2 : Sum  Orientation=left  Inputs=|++  OutDataType=sfix(16)  OutScaling=2^0
  Sum3 : Sum  Orientation=left  Inputs=+-  OutDataType=sfix(16)  OutScaling=2^0
  Irqref : Outport  Orientation=left
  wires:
  -1/(sqrt(3)*Vpp)/1 -> Sum2/1
  Integrator2/1 -> Sum2/2
  Sum2/1 -> Irqref/1
  Qref/1 -> Sum3/1
  Q/1 -> Sum3/2
  Sum3/1 -> Gain6/1, -1/(sqrt(3)*Vpp)/1
  Gain6/1 -> Integrator2/1

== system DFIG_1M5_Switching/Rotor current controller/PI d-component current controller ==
  Ird : Inport  Orientation=left  OutDataType=sfix(16)  OutScaling=2^0
  Irdref : Inport  Orientation=left  Port=2  OutDataType=sfix(16)  OutScaling=2^0
  Gain3 : Gain  Orientation=left  Gain=kp_i  ParameterDataType=sfix(16)  ParameterScaling=2^0  OutDataType=sfix(16)  OutScaling=2^0
  Gain4 : Gain  Orientation=left  Gain=ki_i  ParameterDataType=sfix(16)  ParameterScaling=2^0  OutDataType=sfix(16)  OutScaling=2^0
  Integrator1 : Integrator  Orientation=left
  Sum4 : Sum  Orientation=left  Inputs=+-  OutDataType=sfix(16)  OutScaling=2^0
  Sum5 : Sum  Orientation=left  Inputs=|++  OutDataType=sfix(16)  OutScaling=2^0
  Vrd : Outport  Orientation=left
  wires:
  Integrator1/1 -> Sum5/2
  Ird/1 -> Sum4/2
  Irdref/1 -> Sum4/1
  Sum5/1 -> Vrd/1
  Sum4/1 -> Gain4/1, Gain3/1
  Gain4/1 -> Integrator1/1
  Gain3/1 -> Sum5/1

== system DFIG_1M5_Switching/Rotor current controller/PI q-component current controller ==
  Irqref : Inport  Orientation=left  OutDataType=sfix(16)  OutScaling=2^0
  Irq : Inport  Orientation=left  Port=2  OutDataType=sfix(16)  OutScaling=2^0
  Integrator1 : Integrator  Orientation=left
  Ki : Gain  Orientation=left  Gain=ki_i  ParameterDataType=sfix(16)  ParameterScaling=2^0  OutDataType=sfix(16)  OutScaling=2^0
  Kp : Gain  Orientation=left  Gain=kp_i  ParameterDataType=sfix(16)  ParameterScaling=2^0  OutDataType=sfix(16)  OutScaling=2^0
  Sum : Sum  Orientation=left  OutDataType=sfix(16)  OutScaling=2^0
  Sum1 : Sum  Orientation=left  Inputs=+-  OutDataType=sfix(16)  OutScaling=2^0
  Vrq : Outport  Orientation=left
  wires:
  Sum1/1 -> Ki/1, Kp/1
  Sum/1 -> Vrq/1
  Irq/1 -> Sum1/2
  Irqref/1 -> Sum1/1
  Integrator1/1 -> Sum/2
  Ki/1 -> Integrator1/1
  Kp/1 -> Sum/1

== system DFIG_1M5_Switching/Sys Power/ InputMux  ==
  In1 : Inport  OutDataType=sfix(16)  OutScaling=2^0
  In2 : Inport  Port=2  OutDataType=sfix(16)  OutScaling=2^0
  In3 : Inport  Port=3  OutDataType=sfix(16)  OutScaling=2^0
  Convert1 : DataTypeConversion  OutDataType=sfix(16)  OutScaling=2^0
  Convert2 : DataTypeConversion  OutDataType=sfix(16)  OutScaling=2^0
  Convert3 : DataTypeConversion  OutDataType=sfix(16)  OutScaling=2^0
  Mux : Mux  Inputs=3
  Out : Outport  OutDataType=sfix(16)  OutScaling=2^0
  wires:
  Mux/1 -> Out/1
  In1/1 -> Convert1/1
  In2/1 -> Convert2/1
  In3/1 -> Convert3/1
  Convert1/1 -> Mux/1
  Convert2/1 -> Mux/2
  Convert3/1 -> Mux/3

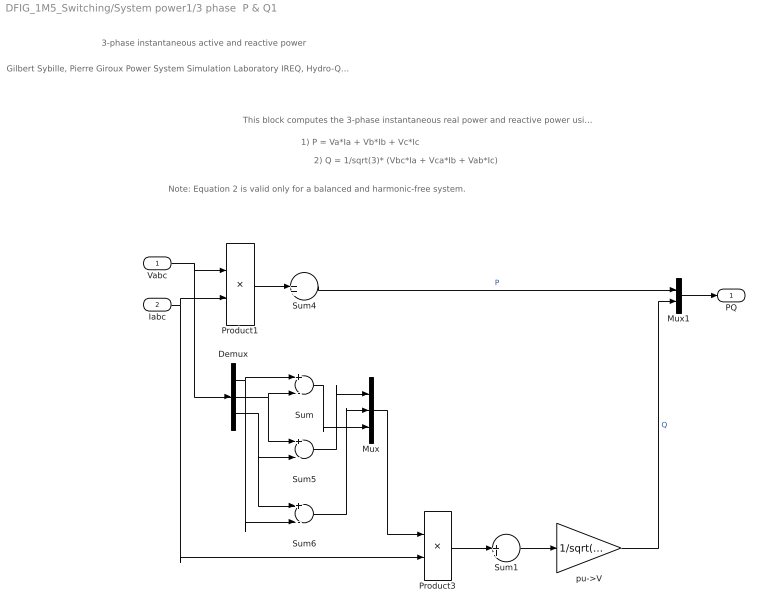
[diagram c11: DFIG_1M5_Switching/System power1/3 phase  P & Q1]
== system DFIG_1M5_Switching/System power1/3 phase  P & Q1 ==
  note: Gilbert Sybille, Pierre Giroux Power System Simulation Laboratory IREQ, Hydro-Quebc
  note: 3-phase instantaneous active and reactive power
  note: Note: Equation 2 is valid only for a balanced and harmonic-free system.
  note: This block computes the 3-phase instantaneous real power and reactive power using the following equations:
  note: 2) Q = 1/sqrt(3)* (Vbc*Ia + Vca*Ib + Vab*Ic)
  note: 1) P = Va*Ia + Vb*Ib + Vc*Ic
  Vabc : Inport  PortDimensions=3  OutDataType=sfix(16)  OutScaling=2^0
  Iabc : Inport  Port=2  PortDimensions=3  OutDataType=sfix(16)  OutScaling=2^0
  Demux : Demux  Outputs=3
  Mux : Mux  Inputs=3
  Mux1 : Mux  Inputs=2
  Product1 : Product  OutDataType=sfix(16)  OutScaling=2^0
  Product3 : Product  OutDataType=sfix(16)  OutScaling=2^0
  Sum : Sum  Inputs=+-  OutDataType=sfix(16)  OutScaling=2^0
  Sum1 : Sum  Inputs=1  OutDataType=sfix(16)  OutScaling=2^0
  Sum4 : Sum  Inputs=1  OutDataType=sfix(16)  OutScaling=2^0
  Sum5 : Sum  Inputs=+-  OutDataType=sfix(16)  OutScaling=2^0
  Sum6 : Sum  Inputs=+-  OutDataType=sfix(16)  OutScaling=2^0
  pu->V : Gain  Gain=1/sqrt(3)  ParameterDataType=sfix(16)  ParameterScaling=2^0  OutDataType=sfix(16)  OutScaling=2^0
  PQ : Outport  OutDataType=sfix(16)  OutScaling=2^0
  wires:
  Mux1/1 -> PQ/1
  pu->V/1 -> Mux1/2  "Q"
  Mux/1 -> Product3/1
  Sum6/1 -> Mux/2
  Sum5/1 -> Mux/1
  Sum/1 -> Mux/3
  Demux/3 -> Sum6/1, Sum5/2
  Demux/2 -> Sum5/1, Sum/2
  Demux/1 -> Sum6/2, Sum/1
  Sum4/1 -> Mux1/1  "P"
  Iabc/1 -> Product3/2, Product1/2
  Vabc/1 -> Demux/1, Product1/1
  Product1/1 -> Sum4/1
  Product3/1 -> Sum1/1
  Sum1/1 -> pu->V/1

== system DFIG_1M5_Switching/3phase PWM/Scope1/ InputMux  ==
  In1 : Inport  OutDataType=sfix(16)  OutScaling=2^0
  Convert1 : DataTypeConversion  OutDataType=sfix(16)  OutScaling=2^0
  Mux : Mux  Inputs=1
  Out : Outport  OutDataType=sfix(16)  OutScaling=2^0
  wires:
  Convert1/1 -> Mux/1
  In1/1 -> Convert1/1
  Mux/1 -> Out/1

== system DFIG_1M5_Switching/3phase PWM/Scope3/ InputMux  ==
  In1 : Inport  OutDataType=sfix(16)  OutScaling=2^0
  Convert1 : DataTypeConversion  OutDataType=sfix(16)  OutScaling=2^0
  Mux : Mux  Inputs=1
  Out : Outport  OutDataType=sfix(16)  OutScaling=2^0
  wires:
  Mux/1 -> Out/1
  In1/1 -> Convert1/1
  Convert1/1 -> Mux/1
